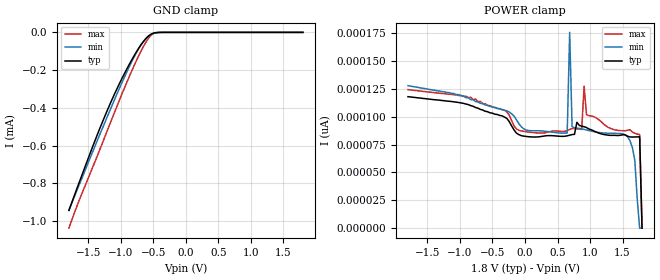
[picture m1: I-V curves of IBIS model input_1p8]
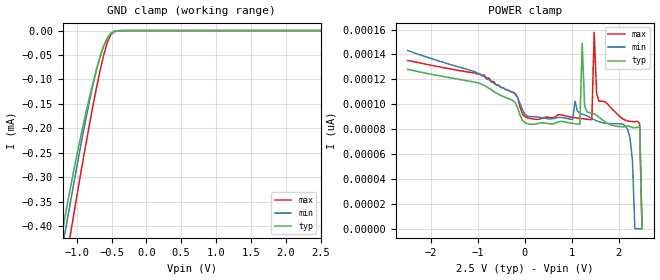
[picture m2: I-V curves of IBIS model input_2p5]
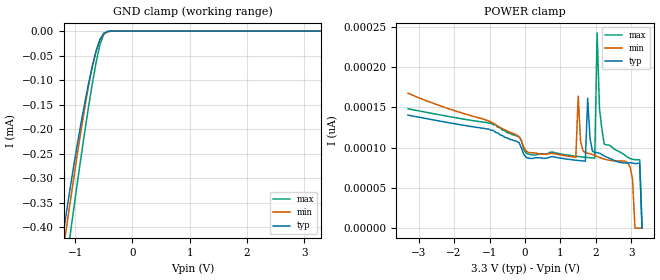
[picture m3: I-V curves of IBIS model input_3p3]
| Texas Instruments Incorporated
| TPUL2G123-Q1 Automotive Dual Monostable-Multivibrator (One-shot)
[IBIS Ver]   3.2
[File name]   tpul2g123-q1.ibs
[File Rev]   1.0
[Date]   09/11/2025
[Source]
| Texas Instruments Incorporated.
| Analog Signal Chain
| Interface - Logic
| 12500 TI Blvd
| Dallas, TX -75243
[Notes] Revision History:
| Rev 1.0: 9/11/2025
| - Initial version of the model
| - Model generated from simulations in SPECTRE
| - Warnings regarding combined Non-monotonicity of various models have been
|   reviewed and considered minor and can be ignored.
| - Model names with a trailing _2p25 contain the model for 2.25V operation.
|   Model names with a trailing _3p3 contain the model for 3.3V operation.
|   Model names with a trailing _5p5 contain the model for 5.5V operation.
[Disclaimer]
| This model is designed as an aid for customers of Texas Instruments.
| TI and its licensors and suppliers make no warranties, either expressed
| or implied, with respect to this  model, including the warranties of
| merchantability or fitness for a particular purpose. The model is
| provided solely on an "as is" basis. The entire risk as to its quality
| and performance is with the customer.
| This model is subject to change without notice. Texas Instruments
| Incorporated is not responsible for updating this model.
[Copyright]
 (C) Copyright 2025 Texas Instruments Incorporated. All rights reserved.
|  Component TPUL2G123PW 16-Pin TSSOP - PW package
[Component]   TPUL2G123PW
[Manufacturer]   Texas Instruments, Inc.
[Package]   |16 TSSOP - PW package
|   typ   min   max
R_pkg   0.045   0.038   0.051
L_pkg   2.593nH   2.447nH   3.080nH
C_pkg   0.281pF   0.243pF   0.377pF
[Pin]   signal_name   model_name   R_pin   L_pin   C_pin
1   1TN   TPUL_IN   NA   NA   NA
2   1T   TPUL_IN   NA   NA   NA
3   1CLRN   TPUL_IN   NA   NA   NA
4   1QN   TPUL_OUT   NA   NA   NA
5   2Q   TPUL_OUT   NA   NA   NA
6   2C   TPUL_IN   NA   NA   NA
7   2RC   TPUL_IN   NA   NA   NA
8   GND   GND   NA   NA   NA
9   2TN   TPUL_IN   NA   NA   NA
10   2T   TPUL_IN   NA   NA   NA
11   2CLRN   TPUL_IN   NA   NA   NA
12   2QN   TPUL_OUT   NA   NA   NA
13   1Q   TPUL_OUT   NA   NA   NA
14   1C   TPUL_IN   NA   NA   NA
15   1RC   TPUL_IN   NA   NA   NA
16   VCC   POWER   NA   NA   NA
|   Model Selectors
[Model Selector] TPUL_IN
input_1p8   1.8V   Schmitt-trigger input
input_2p5   2.5V   Schmitt-trigger input
input_3p3   3.3V   Schmitt-trigger input
input_5   5V   Schmitt-trigger input
[Model Selector] TPUL_OUT
output_1p8   1.8V   push-pull out
output_2p5   2.5V   push-pull out
output_3p3   3.3V   push-pull out
output_5   5V   push-pull out
| Models and submodels in the file (8): input_1p8 (Input), input_2p5 (Input), input_3p3 (Input), input_5 (Input), output_1p8 (Output), output_2p5 (Output), output_3p3 (Output), output_5 (Output)
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|   Input Models
|   Model input_1p8
[Model] input_1p8
Model_type Input
Polarity   Non-Inverting
Enable   Active-High
Vinl =  0.0V
Vinh =  1.800V
C_comp   59.821fF   54.421fF   69.059fF
[Model Spec]
Vinh   1.800V   1.650V   1.950V
Vinl   0.0V   0.0V   0.0V
[Temperature Range]   27.000   0.125k   -40.000
[Voltage Range]   1.800V   1.650V   1.950V
[GND_clamp]
|Voltage   I(typ)   I(min)   I(max)
-1.8V     -944.4uA   -943.4uA   -1.038mA
-1.652V   -805uA     -816.9uA   -899.5uA
-1.355V   -535.6uA   -566.8uA   -647.4uA
-1.206V   -410.8uA   -444.2uA   -517.8uA
-1.058V   -297uA     -324.5uA   -389uA
-872mV    -170.1uA   -182.8uA   -234.9uA
-724mV    -82.78uA   -84.37uA   -122uA
-612mV    -31.41uA   -31.38uA   -49.88uA
-538mV    -9.886uA   -11.29uA   -15.76uA
-464mV    -1.457uA   -2.735uA   -1.7uA
-390mV    -142.6nA   -465.8nA   -93.99nA
1.8V      0A         0A         0A
[POWER_clamp]
|Voltage   I(typ)   I(min)   I(max)
-1.8V     118.1pA    128pA      124.5pA
-92.78mV  83.98pA    93.83pA    87.84pA
649mV     82.92pA    85.46pA    87.58pA
687mV     83.51pA    175.9pA    88.71pA
724mV     84.07pA    91.24pA    89.43pA
872mV     91.6pA     89.2pA     88.66pA
909mV     91.14pA    88.68pA    127.5pA
946mV     90.37pA    88.16pA    102pA
1.577V    82.64pA    81.98pA    87.93pA
1.689V    81.94pA    60.64pA    85.12pA
1.763V    82.1pA     0A         84.11pA
1.8V      0A         0A         0A
|   Model input_2p5
[Model] input_2p5
Model_type Input
Polarity   Non-Inverting
Enable   Active-High
Vinl =  0.0V
Vinh =  2.500V
C_comp   60.880fF   54.874fF   66.715fF
[Model Spec]
Vinh   2.500V   2.250V   2.750V
Vinl   0.0V   0.0V   0.0V
[Temperature Range]   27.000   0.125k   -40.000
[Voltage Range]   2.500V   2.250V   2.750V
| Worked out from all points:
|   GND clamp passes 1 mA (typ) near -1.86 V on its own axis
[GND_clamp]
|Voltage   I(typ)   I(min)   I(max)
-2.5V     -1.617mA   -1.547mA   -1.792mA
-1.224V   -425.7uA   -459.2uA   -533.9uA
-1.173V   -384.8uA   -417.6uA   -489.2uA
-1.122V   -345.3uA   -376.3uA   -444.8uA
-1.071V   -307.1uA   -335.4uA   -400.7uA
-867mV    -167.1uA   -179.5uA   -231.2uA
-714mV    -77.98uA   -78.96uA   -115.5uA
-612mV    -31.25uA   -31.21uA   -49.92uA
-561mV    -15.24uA   -16.01uA   -24.29uA
-510mV    -5.154uA   -6.854uA   -8.116uA
-357mV    -51.93nA   -189.7nA   -24.34nA
2.5V      0A         0A         0A
[POWER_clamp]
|Voltage   I(typ)   I(min)   I(max)
-2.5V     128pA      143.2pA    135.1pA
1.173V    83.86pA    92.77pA    88.62pA
1.224V    148.9pA    92.05pA    88.37pA
1.276V    98.38pA    91.4pA     88.13pA
1.429V    92.81pA    88.56pA    87.5pA
1.48V     92.16pA    87.52pA    157.7pA
1.582V    89.56pA    85.95pA    102.5pA
2.194V    82.53pA    79.61pA    86.58pA
2.296V    81.25pA    54.52pA    86.07pA
2.347V    81.12pA    0A         85.93pA
2.449V    81.78pA    0A         84.55pA
2.5V      0A         0A         0A
|   Model input_3p3
[Model] input_3p3
Model_type Input
Polarity   Non-Inverting
Enable   Active-High
Vinl =  0.0V
Vinh =  3.300V
C_comp   60.292fF   53.652fF   66.121fF
[Model Spec]
Vinh   3.300V   3.000V   3.600V
Vinl   0.0V   0.0V   0.0V
[Temperature Range]   27.000   0.125k   -40.000
[Voltage Range]   3.300V   3.000V   3.600V
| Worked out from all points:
|   GND clamp passes 1 mA (typ) near -1.86 V on its own axis
[GND_clamp]
|Voltage   I(typ)   I(min)   I(max)
-3.3V     -2.397mA   -2.243mA   -2.693mA
-1.233V   -433.1uA   -466.5uA   -541.6uA
-1.167V   -379.6uA   -412.1uA   -483.3uA
-1.1V     -328.4uA   -358.3uA   -425.4uA
-1.033V   -279.5uA   -305.4uA   -368.2uA
-833mV    -145.9uA   -155.5uA   -204.5uA
-700mV    -70.73uA   -71.18uA   -105.8uA
-633mV    -39.96uA   -39.22uA   -62.34uA
-567mV    -16.64uA   -17.49uA   -26.96uA
-500mV    -4.147uA   -5.627uA   -5.756uA
-367mV    -70.23nA   -274.4nA   -33.98nA
3.3V      0A         0A         0A
[POWER_clamp]
|Voltage   I(typ)   I(min)   I(max)
-3.3V     140.4pA    167.6pA    148.3pA
1.433V    84.38pA    88pA       89.38pA
1.5V      84.06pA    164pA      89.02pA
1.7V      83.18pA    93.61pA    88.04pA
1.767V    161.3pA    92.92pA    87.75pA
1.967V    93.87pA    90.29pA    86.89pA
2.033V    93.67pA    88.99pA    242.5pA
2.1V      93.12pA    87.82pA    148.4pA
2.233V    89.75pA    85.79pA    104.4pA
2.967V    81.32pA    75.6pA     86.42pA
3.233V    80.81pA    0A         84.83pA
3.3V      0A         0A         0A
